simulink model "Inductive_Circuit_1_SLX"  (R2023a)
settings: Solver=ode23s  StartTime=0.0  StopTime=10.0  MaxStep=0.001  RelTol=1e-3
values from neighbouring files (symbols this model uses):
  I_2_0 = 0*A    (= 0)    [Inductive_Circuit_1_SLX_m.m]    (also in Electric_Circuit_02_SLX_m.m; Electric_Circuit_03_SLX_m.m; Electric_Circuit_06_SLX_m.m; Electric_Circuit_08_SLX_m.m)
  I_4_0 = 0*A    (= 0)    [Inductive_Circuit_1_SLX_m.m]    (also in Electric_Circuit_02_SLX_m.m; Electric_Circuit_03_SLX_m.m; Electric_Circuit_04_SLX_m.m; Electric_Circuit_05_SLX_m.m)
  I_6_0 = 0*A    (= 0)    [Inductive_Circuit_1_SLX_m.m]    (also in Electric_Circuit_07_SLX_m.m)
  I_8_0 = 0*A    (= 0)    [Inductive_Circuit_1_SLX_m.m]    (also in Electric_Circuit_02_SLX_m.m; Electric_Circuit_05_SLX_m.m; Electric_Circuit_06_SLX_m.m; Electric_Circuit_07_SLX_m.m)
  L_2 = 0.002*H    (= 0.002)    [Inductive_Circuit_1_EQN.m]    (also in Inductive_Circuit_1_SLX_m.m; Electric_Circuit_02_EQN.m; Electric_Circuit_02_SLX_m.m; Electric_Circuit_03_EQN.m)
  L_4 = 0.002*H    (= 0.002)    [Inductive_Circuit_1_EQN.m]    (also in Inductive_Circuit_1_SLX_m.m; Electric_Circuit_02_EQN.m; Electric_Circuit_02_SLX_m.m; Electric_Circuit_03_EQN.m)
  L_6 = 0.002*H    (= 0.002)    [Inductive_Circuit_1_EQN.m]    (also in Inductive_Circuit_1_SLX_m.m; Electric_Circuit_07_EQN.m; Electric_Circuit_07_SLX_m.m; Hydraulic_Circuit_02_EQN.m = 10)
  R_3 = 100*Ohm    (= 100)    [Inductive_Circuit_1_EQN.m]    (also in Inductive_Circuit_1_SLX_m.m; Electric_Circuit_01_EQN.m; Electric_Circuit_01_SLX_m.m; Electric_Circuit_02_EQN.m)
  R_5 = 100*Ohm    (= 100)    [Inductive_Circuit_1_EQN.m]    (also in Inductive_Circuit_1_SLX_m.m; Electric_Circuit_03_EQN.m; Electric_Circuit_03_SLX_m.m; Electric_Circuit_07_EQN.m)
  R_7 = 100*Ohm    (= 100)    [Inductive_Circuit_1_EQN.m]    (also in Inductive_Circuit_1_SLX_m.m; BIG_EC_Simscape_EQN.m; BIG_EC_Simscape_SLX_m.m; Electric_Circuit_03_EQN.m)
  Ts = Tfin/Nr_Ts_Points    (= 3.02935e-07)    [Inductive_Circuit_1_SLX_m.m]    (also in BIG_EC_Simscape_SLX_m.m = 0.0003; Car_Dumper_SLX_m.m = 0.0022779; Electric_Circuit_01_SLX_m.m = 0.005; Electric_Circuit_02_SLX_m.m = 0.000480145)
  V_1_0 = 10*V    (= 10)    [Inductive_Circuit_1_SLX_m.m]    (also in BIG_EC_Simscape_SLX_m.m; Electric_Circuit_02_SLX_m.m; Electric_Circuit_03_SLX_m.m; Electric_Circuit_04_SLX_m.m)

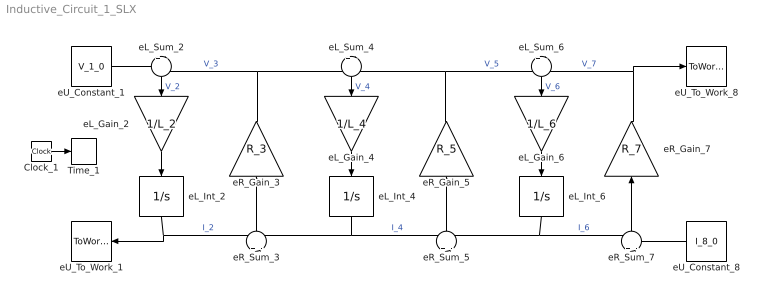
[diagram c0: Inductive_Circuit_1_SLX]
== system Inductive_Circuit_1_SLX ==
  Clock_1 : Clock
  Time_1 : ToWorkspace  VariableName=t  SaveFormat=Timeseries  SampleTime=Ts
  eL_Gain_2 : Gain  Gain=1/L_2  Multiplication=Matrix(K*u)
  eL_Gain_4 : Gain  Gain=1/L_4  Multiplication=Matrix(K*u)
  eL_Gain_6 : Gain  Gain=1/L_6  Multiplication=Matrix(K*u)
  eL_Int_2 : Integrator  InitialCondition=I_2_0
  eL_Int_4 : Integrator  InitialCondition=I_4_0
  eL_Int_6 : Integrator  InitialCondition=I_6_0
  eL_Sum_2 : Sum  Inputs=+|-
  eL_Sum_4 : Sum  Inputs=+|-
  eL_Sum_6 : Sum  Inputs=+|-
  eR_Gain_3 : Gain  Gain=R_3  Multiplication=Matrix(K*u)
  eR_Gain_5 : Gain  Gain=R_5  Multiplication=Matrix(K*u)
  eR_Gain_7 : Gain  Gain=R_7  Multiplication=Matrix(K*u)
  eR_Sum_3 : Sum  Inputs=+|-
  eR_Sum_5 : Sum  Inputs=+|-
  eR_Sum_7 : Sum  Inputs=+|-
  eU_Constant_1 : Constant  Value=V_1_0
  eU_Constant_8 : Constant  Value=I_8_0
  eU_To_Work_1 : ToWorkspace  VariableName=I_1_0  SaveFormat=Timeseries  SampleTime=Ts
  eU_To_Work_8 : ToWorkspace  VariableName=V_8_0  SaveFormat=Timeseries  SampleTime=Ts
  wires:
  eU_Constant_1/1 -> eL_Sum_2/1
  eR_Gain_3/1 -> eL_Sum_2/2, eL_Sum_4/1  "V_3"
  eL_Int_2/1 -> eU_To_Work_1/1, eR_Sum_3/1  "I_2"
  eL_Sum_2/1 -> eL_Gain_2/1  "V_2"
  eL_Gain_2/1 -> eL_Int_2/1
  eL_Int_4/1 -> eR_Sum_3/2, eR_Sum_5/1  "I_4"
  eR_Sum_3/1 -> eR_Gain_3/1
  eR_Gain_5/1 -> eL_Sum_4/2, eL_Sum_6/1  "V_5"
  eL_Sum_4/1 -> eL_Gain_4/1  "V_4"
  eL_Gain_4/1 -> eL_Int_4/1
  eL_Int_6/1 -> eR_Sum_5/2, eR_Sum_7/1  "I_6"
  eR_Sum_5/1 -> eR_Gain_5/1
  eR_Gain_7/1 -> eL_Sum_6/2, eU_To_Work_8/1  "V_7"
  eL_Sum_6/1 -> eL_Gain_6/1  "V_6"
  eL_Gain_6/1 -> eL_Int_6/1
  eU_Constant_8/1 -> eR_Sum_7/2
  eR_Sum_7/1 -> eR_Gain_7/1
  Clock_1/1 -> Time_1/1
